//{{V2}}
FUNCTION FC14
TITLE=Write UInt8 SDO
//*****************************************************************************
//* maxon motor ag
//* R&D
//* all rights reserved
//*****************************************************************************
//* Summary:  Write an UInt8 object via SDO
//*
//* Remarks:
//*
//* Created under: STEP7 REV5.2+SP1
//*****************************************************************************
//* History:
//* 18.05.2004 | INA   first release
//*
//*
//*****************************************************************************


AUTHOR:INA
FAMILY:SDO
NAME:WrtUInt8
VERSION:00.01


VAR_INPUT
       NodeID:BYTE
       Index:DWORD
       SubIndex:DWORD
       ValueIn:BYTE
END_VAR

VAR_OUTPUT
       RET_VAL:BOOL //Done
       Err:BOOL //True = Error detected
       ErrNo:DINT //Error number (CAN or/and VIPA!)
END_VAR

VAR_IN_OUT
END_VAR

VAR_TEMP
       xBusy:BOOL //The write job is not yet completed
       xCanOpenError:DWORD //Return value from SDO transfer
       xRetValue:WORD //VIPA Error
       xValueIn:BYTE
END_VAR
BEGIN

NETWORK
TITLE=
//{{a}}

// SDO Write UInt8

       R    #RET_VAL                     // Done
       R    #Err
       L    0
       T    #ErrNo

       L    #ValueIn
       T    #xValueIn

sfc   :NOP  0


       CALL SFC219
         Request:=TRUE
         Slot_Master:=B#16#00
         NodeID:=#NodeID
         Transfertyp:=B#16#2F            // Write
         Index:=#Index
         Subindex:=#SubIndex
         CanOpenError:=#xCanOpenError
         RetVal:=#xRetValue
         Busy:=#xBusy
         DataBuffer:=P#L 8.0 BYTE 1

       L    1
       U    #xBusy
       SPB  sfc

       S    #RET_VAL

       L    W#16#F021
       L    #xRetValue
       <I
       SPBN ok                           // jump if RetValue lower than 0xF021
       L    W#16#F028
       L    #xRetValue
       >I
       SPB  errV                         // jump if xRetValue between 0xF021 and 0xF028

       L    0
       L    #xCanOpenError
       <>D
       SPB  errC                         // jump if CAN error

ok    :NOP  0
       R    #Err
       SPA  end

errC  :NOP  0                            // CANopen error
       S    #Err
       L    #xCanOpenError
       TAD
       T    #ErrNo
       SPA  end

errV  :NOP  0                            // VIPA error
       S    #Err
       L    0
       T    #ErrNo
       L    #xRetValue                   // RetVal
       T    #ErrNo

end   :NOP  0
END_FUNCTION
